(* Logix 5000 AddOnInstructionDefinition export CFW900_121171; software revision 20.06 *)

ADD_ON_INSTRUCTION CFW900_121171   (* revision 1.0, ExecutePrescan *)
// 121/171 CIP Extended Speed
// AOI with Parameters
// Help:
// Drive setup as follows:
// C9.5.1 = 121/171
// C9.5.2 = 1
// C9.5.3 = 8
// C9.5.4 = 1
// C9.5.5 = 8
// C9.2.1.1 - 3
// C9.2.1.2 - 7
// C9.2.1.3 - 5
// C9.2.1.4 - 60
// C9.2.1.5 - USER DEFINED
// C9.2.1.6 - USER DEFINED
// C9.2.1.7 - USER DEFINED
// C9.2.1.8 - USER DEFINED
// C9.2.2.2 - 100
// C9.2.2.3 - 101
// C9.2.2.4 - USER DEFINED
// C9.2.2.5 - USER DEFINED
// C9.2.2.6 - USER DEFINED
// C9.2.2.7 - USER DEFINED
// C9.2.2.8- USER DEFINED
// C4.1.1 - Ethernet
// C4.2.2.1 - Ethernet
// C4.2.2.2 - Ethernet
// C4.2.2.3 - Ethernet
// C4.2.2.4 - Ethernet
// C4.3.1.2.1 - Keypad
// C4.3.1.2.2 - Ethernet
VAR_INPUT
   ConnectionFaulted : BOOL; {required}   // From CFW900
END_VAR
VAR_IN_OUT
   Inputs : INT[10]; {required}   // Input Assembly From CFW900
   Outputs : INT[10]; {required}   // Output Assembly To CFW900
END_VAR
VAR_INPUT
   Run_Fwd : BOOL; {visible}   // 1 = Run Fwd 0 = Stop
   Run_Rev : BOOL; {visible}   // 1 = Run Rev 0 = Stop
   Fault_Reset : BOOL; {visible}   // 1 = Fault Reset 0 = No action
   NetCtrl : BOOL := 1; {visible}   // 1 = Remote (PLC) Control 0 = Local (HMI) Control
   NetRef : BOOL := 1; {visible}   // 1 = Speed Reference is sent via network 0 = Speed Reference is not being sent via network
   Speed_Reference : INT; {required}   // Speed Setpoint (RPM)
END_VAR
VAR_OUTPUT
   RealSpeed : INT; {access Read Only, visible}   // Current Speed (RPM)
   Connection_Ready : BOOL; {access None, visible}   // Indicates that CFW900 connection is not in a faulted state
   Connection_Faulted : BOOL; {access Read Only, visible}   // Connection is interrupted status bit
   sts_Drv_nrdy : BOOL; {access None, visible}   // 1 = Drive not ready latched until no run cmd given
   Faulted : BOOL; {access Read Only, visible}
   Running_Fwd : BOOL; {access Read Only, visible}   // 1 = CFW900 Running 0 = CFW900 Stopped
   Running_Rev : BOOL; {access Read Only, visible}   // 1 = Motor is rotating 0 = Motor is not rotating
   Warning : BOOL; {access Read Only, visible}   // 1 = drive is in alarm condition 0 = drive is not in alarm condition
   Ready : BOOL; {access Read Only, visible}   // 1 = Drive is ready to operate (states Ready, Enabled or Stopping) 0 = Drive is not ready to operate
   Ctrl_from_net : BOOL; {access Read Only, visible}   // 1 = drive is controlled remotely (PLC) 0 = drive is controlled locally (HMI)
   Ref_from_net : BOOL; {access Read Only, visible}   // 1 = using speed/torque reference received via network 0 = speed/torque reference received via network is disregarded
   At_reference : BOOL; {access Read Only, visible}   // 1 = drive has reached the programmed speed 0 = drive has not yet reached the programmed speed
END_VAR
VAR_INPUT
   cfg_FailToStartDelay : DINT; {access None, visible}
   cfg_FailToStopDelay : DINT; {access None, visible}
END_VAR
VAR_OUTPUT
   FailedToStart : BOOL; {access Read Only, visible}   // Indicates Drive Failed to Start
   FailedToStop : BOOL; {access None, visible}   // Indicates Drive Failed to stop in the time allotted
   Drive_Status : INT; {access Read Only, visible}   // 0 = Non-Existent 1= Startup 2 = Not Ready 3 = Ready 4 = Enabled 5 = Stopping 6 = Fault Stop 7 = Faulted
   val_OutputVoltage : REAL; {access Read Only, visible}
   val_OutputCurrent : REAL; {access Read Only, visible}
   val_OutputFreq : REAL; {access Read Only, visible}
   val_FaultCode : DINT; {access Read Only, visible}
END_VAR
VAR_INPUT
   set_Accel : REAL := 10.0; {required}   // Acceleration Ramp setpoint (0.1-999.9) in seconds
   set_Decel : REAL := 10.0; {required}   // Deceleration Ramp setpoint (0.1-999.9) in seconds
END_VAR
VAR
   FailToStart : TIMER; {access None}
   Wrk_Run1 : BOOL; {access None}   // Internal bit to signal run1
   Wrk_Run2 : BOOL; {access None}   // Internal bit to signal run2
   FailToStop : TIMER; {access None}
   TempReal : REAL; {access None}
   TempDINT : DINT; {access None}
END_VAR

ROUTINE Logic   (* ladder *)
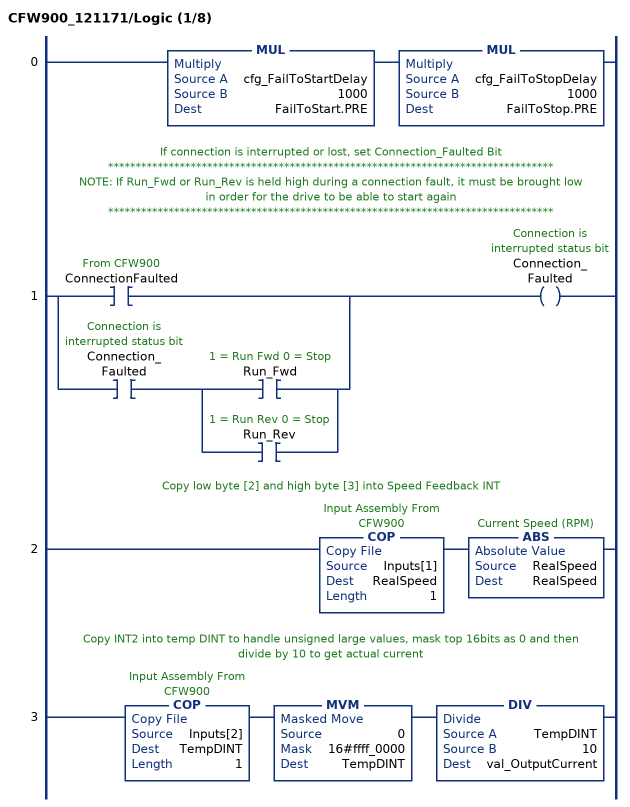
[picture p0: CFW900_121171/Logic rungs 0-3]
   0: MUL(cfg_FailToStartDelay,1000,FailToStart.PRE)MUL(cfg_FailToStopDelay,1000,FailToStop.PRE);
   // If connection is interrupted or lost, set Connection_Faulted Bit
   // *********************************************************************************
   // NOTE: If Run_Fwd or Run_Rev is held high during a connection fault, it must be brought low
   // in order for the drive to be able to start again
   // *********************************************************************************
   1: [XIC(ConnectionFaulted) ,XIC(Connection_Faulted) [XIC(Run_Fwd) ,XIC(Run_Rev) ] ]OTE(Connection_Faulted);
   // Copy low byte [2] and high byte [3] into Speed Feedback INT
   2: COP(Inputs[1],RealSpeed,1)ABS(RealSpeed,RealSpeed);
   // Copy INT2 into temp DINT to handle unsigned large values, mask top 16bits as 0 and then divide by 10 to get actual current
   3: COP(Inputs[2],TempDINT,1)MVM(0,16#ffff_0000,TempDINT)DIV(TempDINT,10,val_OutputCurrent);
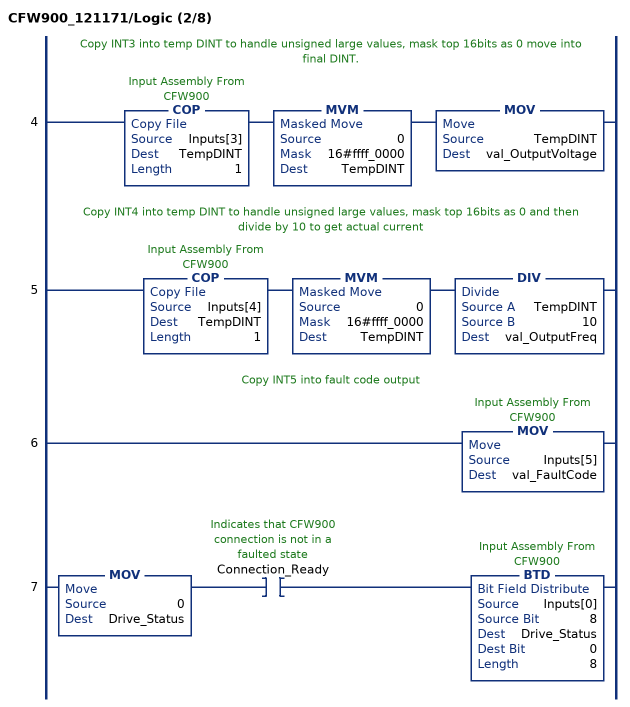
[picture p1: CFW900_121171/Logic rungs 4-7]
   // Copy INT3 into temp DINT to handle unsigned large values, mask top 16bits as 0 move into final DINT.
   4: COP(Inputs[3],TempDINT,1)MVM(0,16#ffff_0000,TempDINT)MOV(TempDINT,val_OutputVoltage);
   // Copy INT4 into temp DINT to handle unsigned large values, mask top 16bits as 0 and then divide by 10 to get actual current
   5: COP(Inputs[4],TempDINT,1)MVM(0,16#ffff_0000,TempDINT)DIV(TempDINT,10,val_OutputFreq);
   // Copy INT5 into fault code output
   6: MOV(Inputs[5],val_FaultCode);
   7: MOV(0,Drive_Status)XIC(Connection_Ready)BTD(Inputs[0],8,Drive_Status,0,8);
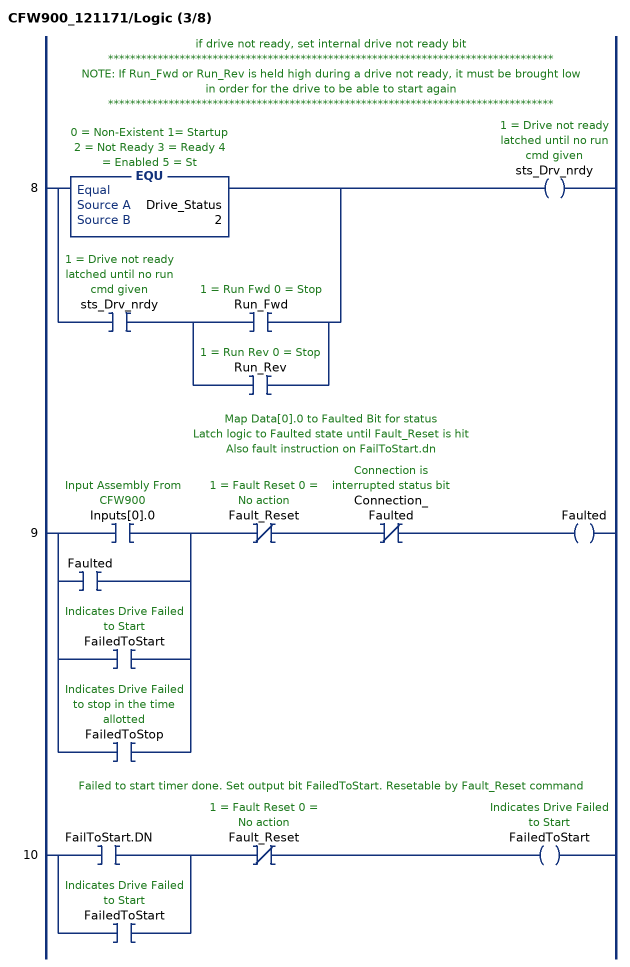
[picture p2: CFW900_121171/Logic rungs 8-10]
   // if drive not ready, set internal drive not ready bit
   // *********************************************************************************
   // NOTE: If Run_Fwd or Run_Rev is held high during a drive not ready, it must be brought low
   // in order for the drive to be able to start again
   // *********************************************************************************
   8: [EQU(Drive_Status,2) ,XIC(sts_Drv_nrdy) [XIC(Run_Fwd) ,XIC(Run_Rev) ] ]OTE(sts_Drv_nrdy);
   // Map Data[0].0 to Faulted Bit for status
   // Latch logic to Faulted state until Fault_Reset is hit
   // Also fault instruction on FailToStart.dn
   9: [XIC(Inputs[0].0) ,XIC(Faulted) ,XIC(FailedToStart) ,XIC(FailedToStop) ]XIO(Fault_Reset)XIO(Connection_Faulted)OTE(Faulted);
   // Failed to start timer done. Set output bit FailedToStart. Resetable by Fault_Reset command
   10: [XIC(FailToStart.DN) ,XIC(FailedToStart) ]XIO(Fault_Reset)OTE(FailedToStart);
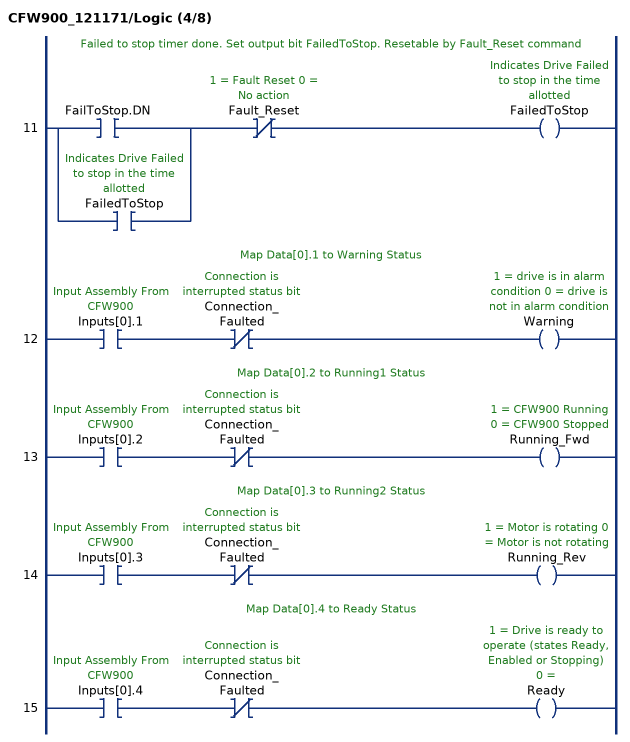
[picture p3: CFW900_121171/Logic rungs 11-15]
   // Failed to stop timer done. Set output bit FailedToStop. Resetable by Fault_Reset command
   11: [XIC(FailToStop.DN) ,XIC(FailedToStop) ]XIO(Fault_Reset)OTE(FailedToStop);
   // Map Data[0].1 to Warning Status
   12: XIC(Inputs[0].1)XIO(Connection_Faulted)OTE(Warning);
   // Map Data[0].2 to Running1 Status
   13: XIC(Inputs[0].2)XIO(Connection_Faulted)OTE(Running_Fwd);
   // Map Data[0].3 to Running2 Status
   14: XIC(Inputs[0].3)XIO(Connection_Faulted)OTE(Running_Rev);
   // Map Data[0].4 to Ready Status
   15: XIC(Inputs[0].4)XIO(Connection_Faulted)OTE(Ready);
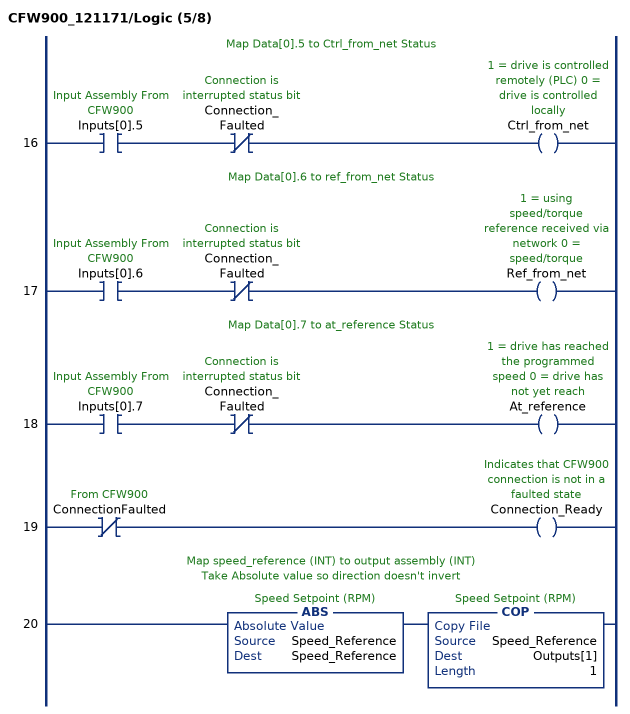
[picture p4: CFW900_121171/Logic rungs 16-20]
   // Map Data[0].5 to Ctrl_from_net Status
   16: XIC(Inputs[0].5)XIO(Connection_Faulted)OTE(Ctrl_from_net);
   // Map Data[0].6 to ref_from_net Status
   17: XIC(Inputs[0].6)XIO(Connection_Faulted)OTE(Ref_from_net);
   // Map Data[0].7 to at_reference Status
   18: XIC(Inputs[0].7)XIO(Connection_Faulted)OTE(At_reference);
   19: XIO(ConnectionFaulted)OTE(Connection_Ready);
   // Map speed_reference (INT) to output assembly (INT)
   // Take Absolute value so direction doesn't invert
   20: ABS(Speed_Reference,Speed_Reference)COP(Speed_Reference,Outputs[1],1);
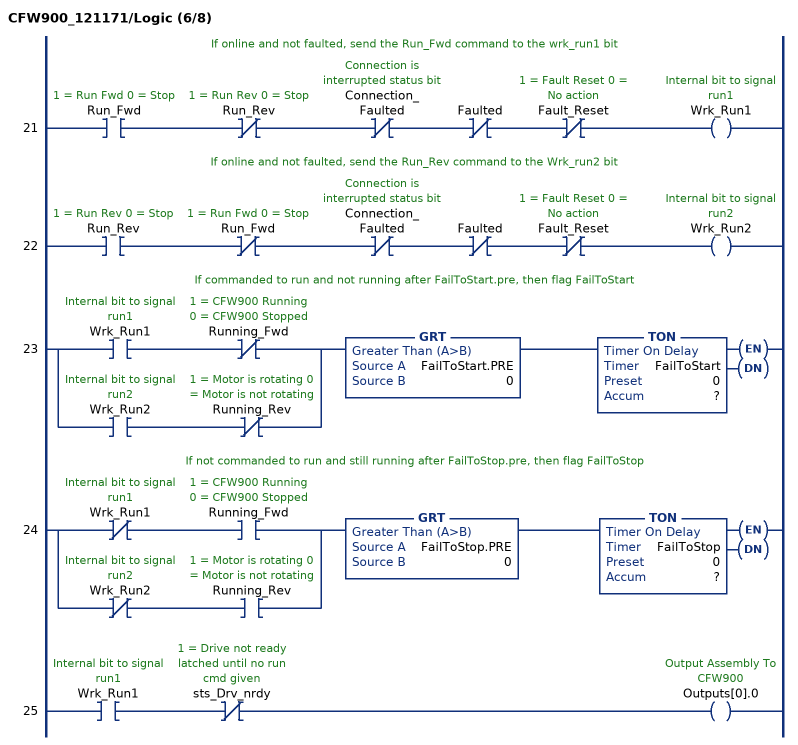
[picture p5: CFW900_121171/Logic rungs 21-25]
   // If online and not faulted, send the Run_Fwd command to the wrk_run1 bit
   21: XIC(Run_Fwd)XIO(Run_Rev)XIO(Connection_Faulted)XIO(Faulted)XIO(Fault_Reset)OTE(Wrk_Run1);
   // If online and not faulted, send the Run_Rev command to the Wrk_run2 bit
   22: XIC(Run_Rev)XIO(Run_Fwd)XIO(Connection_Faulted)XIO(Faulted)XIO(Fault_Reset)OTE(Wrk_Run2);
   // If commanded to run and not running after FailToStart.pre, then flag FailToStart
   23: [XIC(Wrk_Run1) XIO(Running_Fwd) ,XIC(Wrk_Run2) XIO(Running_Rev) ]GRT(FailToStart.PRE,0)TON(FailToStart,?,?);
   // If not commanded to run and still running after FailToStop.pre, then flag FailToStop
   24: [XIO(Wrk_Run1) XIC(Running_Fwd) ,XIO(Wrk_Run2) XIC(Running_Rev) ]GRT(FailToStop.PRE,0)TON(FailToStop,?,?);
   25: XIC(Wrk_Run1)XIO(sts_Drv_nrdy)OTE(Outputs[0].0);
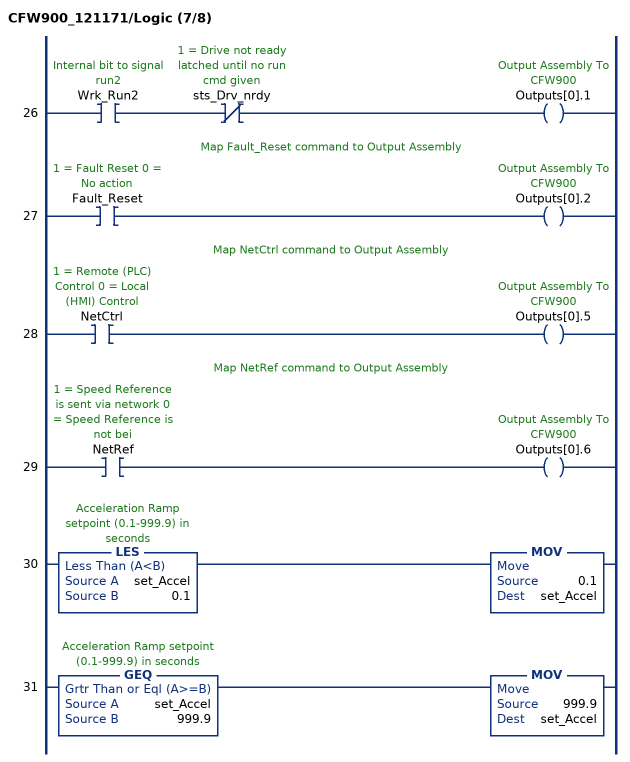
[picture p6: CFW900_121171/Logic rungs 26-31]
   26: XIC(Wrk_Run2)XIO(sts_Drv_nrdy)OTE(Outputs[0].1);
   // Map Fault_Reset command to Output Assembly
   27: XIC(Fault_Reset)OTE(Outputs[0].2);
   // Map NetCtrl command to Output Assembly
   28: XIC(NetCtrl)OTE(Outputs[0].5);
   // Map NetRef command to Output Assembly
   29: XIC(NetRef)OTE(Outputs[0].6);
   30: LES(set_Accel,0.1)MOV(0.1,set_Accel);
   31: GEQ(set_Accel,999.9)MOV(999.9,set_Accel);
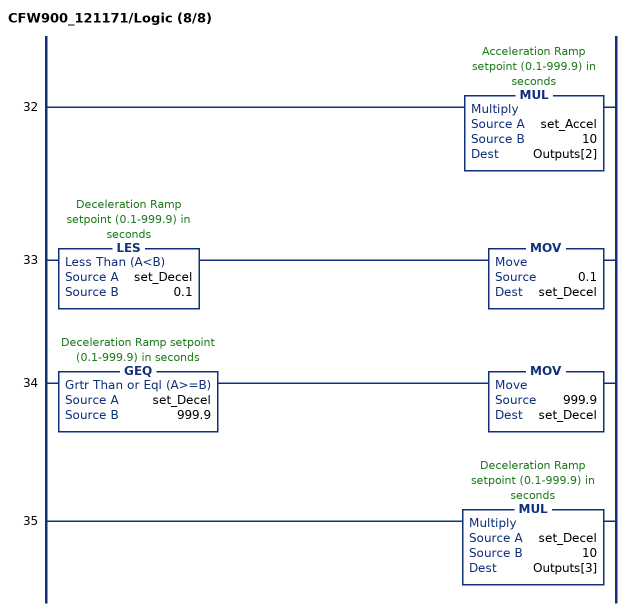
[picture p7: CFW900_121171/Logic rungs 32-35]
   32: MUL(set_Accel,10,Outputs[2]);
   33: LES(set_Decel,0.1)MOV(0.1,set_Decel);
   34: GEQ(set_Decel,999.9)MOV(999.9,set_Decel);
   35: MUL(set_Decel,10,Outputs[3]);
END_ROUTINE

ROUTINE Prescan   (* ladder *)
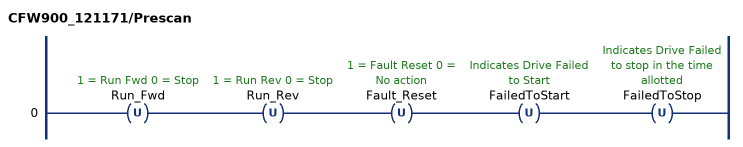
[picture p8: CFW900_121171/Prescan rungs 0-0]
   0: OTU(Run_Fwd)OTU(Run_Rev)OTU(Fault_Reset)OTU(FailedToStart)OTU(FailedToStop);
END_ROUTINE
END_ADD_ON_INSTRUCTION
